(* Logix 5000 DataType export R8AI8DIDO_Seneca_OutData; software revision 35.00 *)

TYPE R8AI8DIDO_Seneca_OutData :   // User Define Data Out Type for Seneca R-8AI-8DIDO-2-E Device
STRUCT
   DOUT1 : BOOL;   // Digital Output1
   DOUT2 : BOOL;   // Digital Output2
   DOUT3 : BOOL;   // Digital Output3
   DOUT4 : BOOL;   // Digital Output4
   DOUT5 : BOOL;   // Digital Output5
   DOUT6 : BOOL;   // Digital Output6
   DOUT7 : BOOL;   // Digital Output7
   DOUT8 : BOOL;   // Digital Output8
   CMD : INT;   // Command Register
   CMD_AUX : UDINT;   // Command Auxiliar
END_STRUCT
END_TYPE
